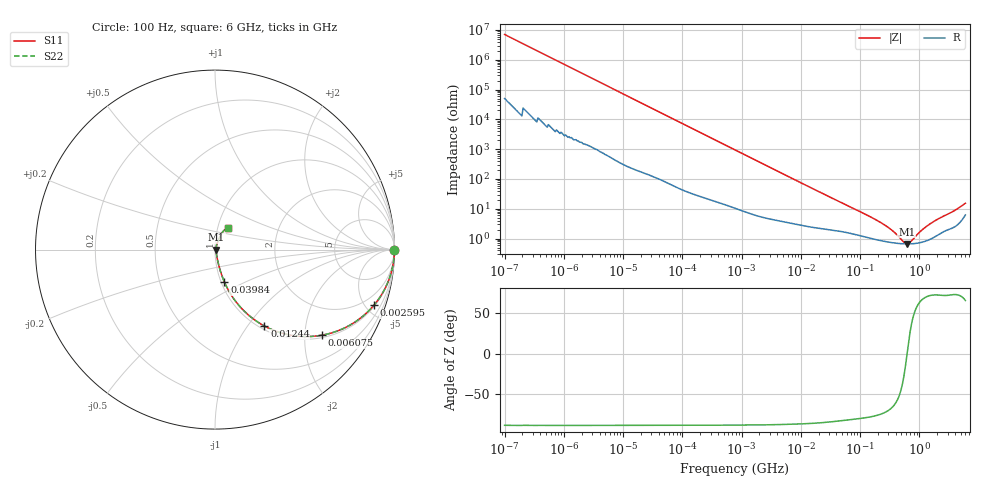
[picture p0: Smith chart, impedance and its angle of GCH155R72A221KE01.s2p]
!Murata Part Number: GCH155R72A221KE01
!These Parameters are Measured in Series Mode Connection
!Data Generated on Mar 13, 2026
!  o--ll--o
!Port1  Port2
!  o------o
!Operation Temp=25[degC], DC Bias Voltage=0[V]
!Freq. Start=100[Hz] Stop=6[GHz] 401[Steps]
# Hz S RI R 50
!Freq.(Hz) S11(Real) S11(Imag) S21(Real) S21(Imag) S12(Real) S12(Imag) S22(Real) S22(Imag)
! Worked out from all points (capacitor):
!   401 points, 100 Hz to 6 GHz, reference 50 ohm
!   read as one part in series: C = 224 pF near 109 Hz
!   lowest |Z| = 662 mohm at 611.6 MHz (marker M1)
!   series resonance near 622.4 MHz, so ESL is about 290 pH
!   S11 on the Smith chart (normalised r, x): 100 Hz: open; 2.595 MHz: 1.10, -5.68; 6.075 MHz: 1.07, -2.44; 12.44 MHz: 1.05, -1.20; 39.84 MHz: 1.04, -0.39; 6 GHz: 1.12, +0.28
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100  1 -1.41e-05  1e-07 1.41e-05  1e-07 1.41e-05  1 -1.41e-05
686  1 -9.6e-05  4e-07 9.6e-05  4e-07 9.6e-05  1 -9.6e-05
2008  1 -0.00028  1.4e-06 0.00028  1.4e-06 0.00028  1 -0.00028
40335  0.9999 -0.00558  6.21e-05 0.00558  6.21e-05 0.00558  0.9999 -0.00558
241822  0.9986 -0.0332  0.00136 0.0332  0.00136 0.0332  0.9986 -0.0332
774597  0.9878 -0.1044  0.0122 0.1044  0.0122 0.1044  0.9878 -0.1044
2594782  0.8856 -0.3099  0.1144 0.3099  0.1144 0.3099  0.8856 -0.3099
3882480  0.7788 -0.4045  0.2212 0.4045  0.2212 0.4045  0.7788 -0.4045
6075234  0.5964 -0.4768  0.4036 0.4768  0.4036 0.4768  0.5964 -0.4768
8692127  0.4266 -0.4776  0.5734 0.4776  0.5734 0.4776  0.4266 -0.4776
1.243624e7  0.2751 -0.4256  0.7249 0.4256  0.7249 0.4256  0.2751 -0.4256
1.555665e7  0.2011 -0.3769  0.7989 0.3769  0.7989 0.3769  0.2011 -0.3769
2.434276e7  0.1038 -0.2731  0.8962 0.2731  0.8962 0.2731  0.1038 -0.2731
3.983537e7  0.052 -0.1795  0.948 0.1795  0.948 0.1795  0.052 -0.1795
1.526266e8  0.0125 -0.0504  0.9875 0.0504  0.9875 0.0504  0.0125 -0.0504
3.124326e8  0.00789 -0.0206  0.9921 0.0206  0.9921 0.0206  0.00789 -0.0206
5.346885e8  0.00663 -0.00432  0.9934 0.00432  0.9934 0.00432  0.00663 -0.00432
6.11557e8  0.00656 -0.000496  0.9934 0.000496  0.9934 0.000496  0.00656 -0.000496
6.994765e8  0.0066 0.00335  0.9934 -0.00335  0.9934 -0.00335  0.0066 0.00335
1.046602e9  0.00751 0.0156  0.9925 -0.0156  0.9925 -0.0156  0.00751 0.0156
1.565993e9  0.0105 0.0303  0.9895 -0.0303  0.9895 -0.0303  0.0105 0.0303
6e9  0.0745 0.1225  0.9255 -0.1225  0.9255 -0.1225  0.0745 0.1225
